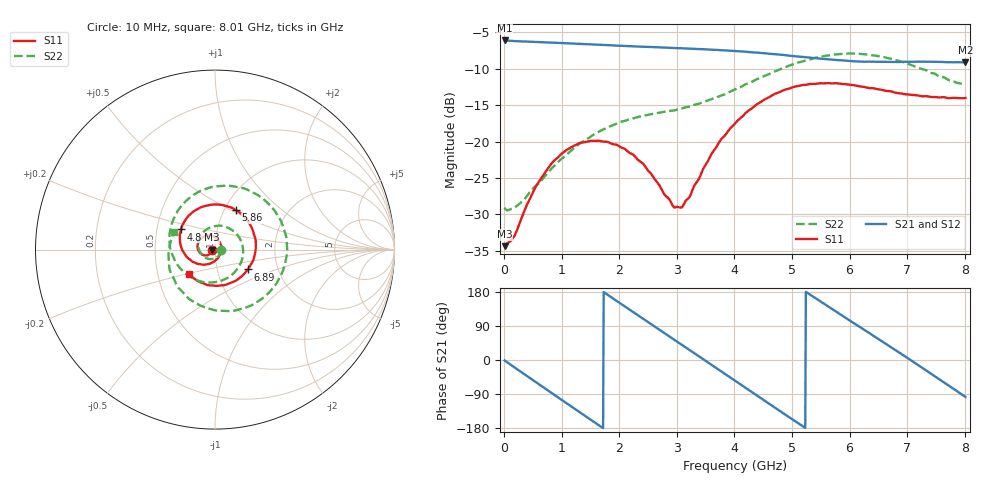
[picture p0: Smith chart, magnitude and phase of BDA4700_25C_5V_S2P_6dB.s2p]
!Agilent Technologies,E5071B,MY42404982,A.09.10
!Date: Mon Oct 20 13:28:56 2025
!Data & Calibration Information:
!Freq	S11:SOLT2(ON)	S21:SOLT2(ON)	S12:SOLT2(ON)	S22:SOLT2(ON)
# Hz S RI R 50
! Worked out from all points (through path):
!   801 points, 10 MHz to 8.01 GHz, reference 50 ohm
!   highest |S21| = -6.11 dB at 10 MHz (marker M1); lowest = -9.1 dB at 8.01 GHz (marker M2)
!   group delay of S21, straight-line fit = 283 ps
!   lowest |S11| = -34.4 dB at 10 MHz (marker M3), VSWR 1.04, Z = 48.1 - j0.0966 ohm
!   |S11| at or under -10 dB: start of sweep to end of sweep
!   |S22| runs from -29.4 to -7.9 dB; largest |S21 - S12| = 0.0038
!   S11 on the Smith chart (normalised r, x): 10 MHz: 0.96, -0.00; 4.8 GHz: 0.67, +0.16; 5.86 GHz: 1.14, +0.53; 6.89 GHz: 1.40, -0.33; 8.01 GHz: 0.72, -0.20
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1e7  -0.0191 -0.001  0.4947 -0.0105  0.4947 -0.0112  0.0351 -0.0029
3.3e8  -0.0248 -0.0196  0.3982 -0.2805  0.3981 -0.2809  0.0219 -0.0325
7.2e8  -0.0527 -0.0328  0.1158 -0.4658  0.1158 -0.466  -0.0243 -0.0532
1.02e9  -0.081 -0.0211  -0.1407 -0.4532  -0.1411 -0.4533  -0.0701 -0.0323
1.35e9  -0.0978 0.0121  -0.3664 -0.2913  -0.3668 -0.2914  -0.0938 0.0318
1.64e9  -0.0897 0.0473  -0.4573 -0.0681  -0.4577 -0.068  -0.0664 0.0958
1.93e9  -0.0618 0.0727  -0.4251 0.1671  -0.4252 0.1675  0.00456 0.1315
2.32e9  -0.0118 0.0742  -0.2147 0.395  -0.2146 0.3951  0.1129 0.0945
2.68e9  0.0256 0.0443  0.0642 0.4393  0.0641 0.4391  0.1568 -0.0142
2.94e9  0.0348 0.00821  0.2516 0.3605  0.2517 0.3599  0.1298 -0.0992
3.09e9  0.0323 -0.0145  0.3368 0.2789  0.3354 0.2797  0.0946 -0.14
3.54e9  -0.0149 -0.072  0.4267 -0.0476  0.4263 -0.0483  -0.0641 -0.1807
4.01e9  -0.111 -0.0736  0.2425 -0.3422  0.2424 -0.3418  -0.2154 -0.0755
4.39e9  -0.1804 -0.00725  -0.0267 -0.4074  -0.0265 -0.4079  -0.2533 0.0877
4.8e9  -0.1892 0.1121  -0.2827 -0.2758  -0.2818 -0.2766  -0.1649 0.2678
5.35e9  -0.0636 0.2406  -0.3686 0.0733  -0.369 0.0726  0.1239 0.3484
5.86e9  0.1178 0.2191  -0.1701 0.3187  -0.1698 0.3186  0.3662 0.1621
6.25e9  0.2099 0.1111  0.0601 0.3482  0.0637 0.3476  0.3886 -0.0856
6.68e9  0.2179 -0.0446  0.2793 0.2145  0.2801 0.2143  0.2255 -0.2969
6.89e9  0.1833 -0.1105  0.3368 0.1019  0.3374 0.1003  0.1012 -0.3411
7.48e9  0.00936 -0.202  0.2577 -0.2408  0.2579 -0.2418  -0.2136 -0.2003
8.01e9  -0.1452 -0.1363  -0.0458 -0.3468  -0.0461 -0.3469  -0.2274 0.1005
